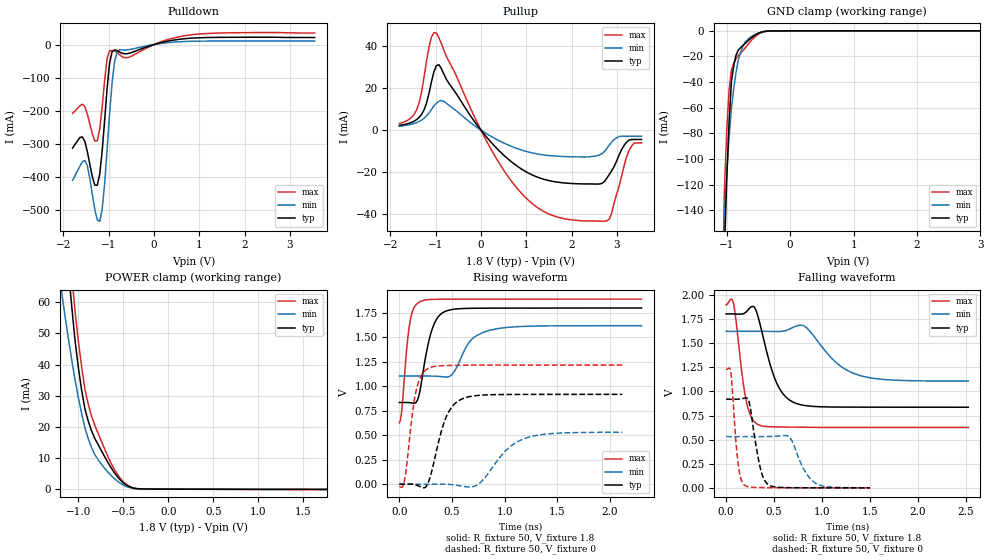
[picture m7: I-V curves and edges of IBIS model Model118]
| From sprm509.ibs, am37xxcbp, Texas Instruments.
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| Model based on original model for BQOMAPGFR50CHYFBPBNOPM_SSBHV
|   Sub model HYFBPBNOPM_V_PU1_1P8
[model]   Model118
|[Input Load]   PU
|[Output Drive]
|Voltage   1.8V
|Mode   I/O
Model_type   I/O
Polarity   Non-Inverting
Enable   Active-Low
Vinl =  0.63
Vinh =  1.17
Cref =  15pF
Rref =  100.0000M
Vref =  0V
Vmeas =  0.9
C_comp   1.661533p   1.48038p   1.850162p
[Model Spec]
Vinl   0.63   0.567   0.6615
Vinh   1.17   1.053   1.2285
[Temperature Range]   25   125   -40
[Voltage Range]   1.8   1.62   1.89
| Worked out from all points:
|   slope of the pulldown table from 0 to 0.27 V, typ, clamps not added: 28.9 ohm
|   slope of the pullup table from 0 to 0.27 V, typ, clamps not added: 39.5 ohm
|   GND clamp passes 1 mA (typ) near -0.45 V on its own axis
|   POWER clamp passes 1 mA (typ) near -0.45 V on its own axis
|   rising waveform, R_fixture 50, V_fixture 1.8: 20-80 % time 112ps typ, 181ps min, 64.9ps max; typ from 0.835 V to 1.8 V
|   rising waveform, R_fixture 50, V_fixture 0: 20-80 % time 147ps typ, 266ps min, 89.5ps max; typ from 0.001 V to 0.918 V
|   falling waveform, R_fixture 50, V_fixture 1.8: 20-80 % time 182ps typ, 323ps min, 101ps max; typ from 1.8 V to 0.836 V
|   falling waveform, R_fixture 50, V_fixture 0: 20-80 % time 95.3ps typ, 154ps min, 58.6ps max; typ from 0.919 V to 0.002 V
[POWER_clamp]
-1.8V     350.2mA    199.8mA    415mA
-1.182V   95.17mA    62.16mA    110.3mA
-1.109V   69.62mA    47.9mA     81.05mA
-1.073V   58.12mA    41.25mA    68.34mA
-1.036V   47.39mA    34.88mA    56.74mA
-1V       38.89mA    29.28mA    47.37mA
-927.3mV  25.68mA    19.62mA    32mA
-890.9mV  21.86mA    16.22mA    27.3mA
-672.7mV  8.613mA    5.512mA    10.52mA
-490.9mV  1.745mA    1.127mA    2.082mA
-309.1mV  68.17uA    54.83uA    85.18uA
1.764V    -96.75uA   -47.78uA   -163.6uA
[Pulldown]
-1.8V     -313.1mA   -410.8mA   -208.2mA
-1.527V   -293.3mA   -350.9mA   -188.2mA
-1.473V   -324.4mA   -367.2mA   -211mA
-1.309V   -425.1mA   -498.2mA   -291.7mA
-1.2V     -391.6mA   -534.5mA   -255.3mA
-1.091V   -227.7mA   -419.3mA   -107mA
-1.036V   -131.1mA   -316mA     -42.16mA
-981.8mV  -55.68mA   -208.4mA   -18.81mA
-872.7mV  -16.14mA   -52.01mA   -19.81mA
-763.6mV  -22.7mA    -15.88mA   -30.69mA
872.7mV   19.66mA    9.937mA    30.15mA
3.545V    21.28mA    10.46mA    34.9mA
[Pullup]
-1.8V     2.19mA     1.826mA    3.106mA
-1.418V   4.982mA    3.55mA     9.585mA
-1.255V   9.598mA    5.591mA    25.18mA
-1.145V   17.5mA     8.127mA    39.43mA
-1.036V   27.75mA    11.5mA     46.22mA
-927.3mV  30.99mA    13.66mA    43.72mA
381.8mV   -9.36mA    -4.816mA   -14.9mA
1.418V    -23.5mA    -11.86mA   -38.93mA
2.618V    -25.57mA   -11.79mA   -43.15mA
2.836V    -20.91mA   -7.019mA   -42.19mA
3.273V    -4.719mA   -2.957mA   -9.576mA
3.545V    -4.444mA   -2.948mA   -6.098mA
[GND_clamp]
-1.8V     -5.203A    -4.842A    -5.388A
-1.073V   -253.8mA   -199.1mA   -208.9mA
-1.036V   -171.9mA   -145.3mA   -123.3mA
-1V       -115.3mA   -111.4mA   -77.09mA
-963.6mV  -71.3mA    -83.17mA   -46.24mA
-927.3mV  -39.92mA   -60.68mA   -30.78mA
-890.9mV  -27.38mA   -45.38mA   -25.55mA
-818.2mV  -14.99mA   -22.62mA   -19.16mA
-781.8mV  -13.18mA   -16.62mA   -17.39mA
-600mV    -4.942mA   -4.119mA   -6.754mA
-309.1mV  -131.5uA   -141.8uA   -204.2uA
3.6V      0A         0A         0A
[Ramp]
dV/dt_f  0.6263622/0.188316n   0.3477626/0.3395936n  0.7960786/0.1036366n
dV/dt_r  0.5729377/0.1495207n  0.3353974/0.2740098n  0.7488204/89.51748p
R_load = 50
[Rising Waveform]
R_fixture = 50
V_fixture = 1.8
V_fixture_min = 1.62
V_fixture_max = 1.89
0s        834.7mV    1.104V     626.4mV
24ps      834.5mV    1.104V     768.7mV
93ps      833.2mV    1.105V     1.605V
126ps     828mV      1.104V     1.769V
192ps     936.5mV    1.104V     1.861V
303ps     1.556V     1.104V     1.886V
438ps     1.766V     1.094V     1.889V
687ps     1.796V     1.48V      1.889V
858ps     1.797V     1.572V     1.889V
2.298ns   1.799V     1.618V     1.889V
[Rising Waveform]
R_fixture = 50
V_fixture = 0
V_fixture_min = 0
V_fixture_max = 0
0s        1.035mV    1.07mV     -21.09mV
54ps      980.6uV    1.173mV    71.35mV
159ps     -6.807mV   847.7uV    954.8mV
264ps     -6.953mV   313.3uV    1.177V
432ps     654mV      1.342mV    1.212V
591ps     869.4mV    -18.28mV   1.215V
750ps     907.1mV    247.7uV    1.217V
1.005ns   916mV      338mV      1.217V
1.185ns   917mV      465.7mV    1.217V
2.115ns   917.9mV    530.2mV    1.217V
[Falling Waveform]
R_fixture = 50
V_fixture = 1.8
V_fixture_min = 1.62
V_fixture_max = 1.89
0s        1.801V     1.62V      1.893V
78ps      1.8V       1.62V      1.905V
210ps     1.822V     1.621V     897.9mV
330ps     1.781V     1.621V     657.9mV
519ps     1.104V     1.619V     632.3mV
696ps     889mV      1.661V     630mV
840ps     850.7mV    1.656V     628.2mV
1.131ns   837.7mV    1.312V     626.8mV
1.38ns    836.5mV    1.168V     626.7mV
2.526ns   835.7mV    1.106V     626.7mV
[Falling Waveform]
R_fixture = 50
V_fixture = 0
V_fixture_min = 0
V_fixture_max = 0
0s        919mV      532.5mV    1.223V
45ps      918.7mV    532mV      1.216V
123ps     919.1mV    532.1mV    266.2mV
192ps     930.1mV    532.2mV    28.99mV
240ps     887.2mV    532.2mV    11.7mV
357ps     202.5mV    532mV      4.963mV
432ps     39.86mV    532.5mV    3.612mV
660ps     4.077mV    527.6mV    2.303mV
942ps     2.452mV    45.05mV    2.097mV
1.5ns     1.936mV    2.712mV    2.037mV
